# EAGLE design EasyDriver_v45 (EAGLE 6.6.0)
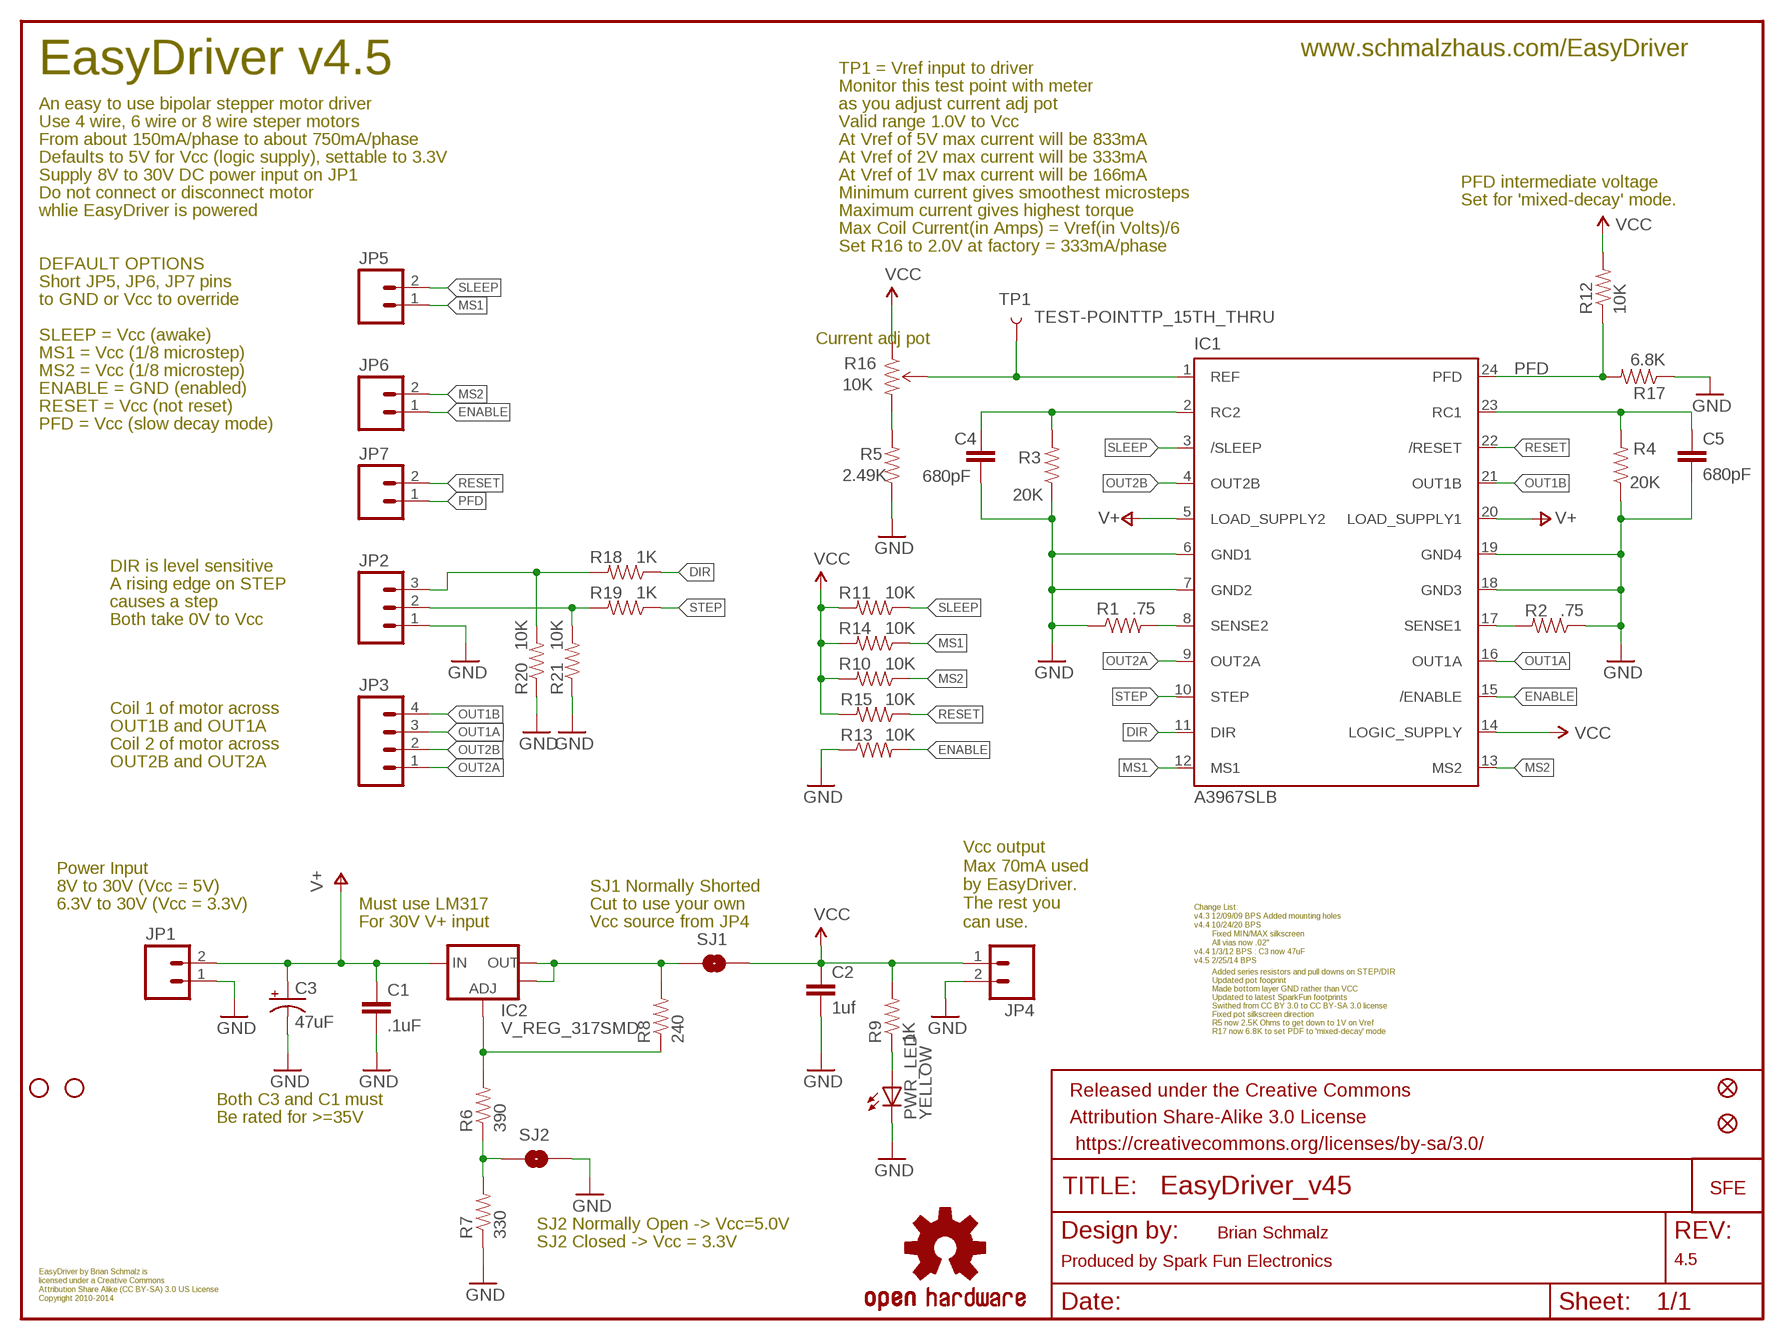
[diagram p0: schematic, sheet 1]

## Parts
C1  .1uF  CAP0603-CAP  [0603-CAP]
C2  1uf  CAP0603-CAP  [0603-CAP]
C3  47uF  CPOL-USD  [PANASONIC_D]
C4  680pF  CAP0603-CAP  [0603-CAP]
C5  680pF  CAP0603-CAP  [0603-CAP]
FID1  FIDUCIAL1X2  [FIDUCIAL-1X2]
FID2  FIDUCIAL1X2  [FIDUCIAL-1X2]
FRAME2  FRAME-LETTER  [CREATIVE_COMMONS]
IC1  A3967SLB  [SO24W]
IC2  V_REG_317SMD  [SOT223]
JP1  M021X02_NO_SILK  [1X02_NO_SILK]
JP2  M031X03_NO_SILK  [1X03_NO_SILK]
JP3  M041X04_NO_SILK  [1X04_NO_SILK]
JP4  M021X02_NO_SILK  [1X02_NO_SILK]
JP5  M021X02_NO_SILK  [1X02_NO_SILK]
JP6  M021X02_NO_SILK  [1X02_NO_SILK]
JP7  M021X02_NO_SILK  [1X02_NO_SILK]
JP8  STAND-OFF  [STAND-OFF]
JP9  STAND-OFF  [STAND-OFF]
LOGO1  OSHW-LOGOS  [OSHW-LOGO-S]
PWR_LED  YELLOW  LED-YELLOW0603  [LED-0603]
R1  .75  RESISTOR0805-RES  [0805]
R2  .75  RESISTOR0805-RES  [0805]
R3  20K  RESISTOR0603  [0603-RES]
R4  20K  RESISTOR0603  [0603-RES]
R5  2.49K  RESISTOR0603  [0603-RES]
R6  390  RESISTOR0603  [0603-RES]
R7  330  RESISTOR0603  [0603-RES]
R8  240  RESISTOR0603  [0603-RES]
R9  1K  RESISTOR0603  [0603-RES]
R10  10K  RESISTOR0603  [0603-RES]
R11  10K  RESISTOR0603  [0603-RES]
R12  10K  RESISTOR0603  [0603-RES]
R13  10K  RESISTOR0603  [0603-RES]
R14  10K  RESISTOR0603  [0603-RES]
R15  10K  RESISTOR0603  [0603-RES]
R16  10K  TRIMPOT3MM-2  [TRIMPOT-3MM-2]
R17  6.8K  RESISTOR0603  [0603-RES]
R18  1K  RESISTOR0603  [0603-RES]
R19  1K  RESISTOR0603  [0603-RES]
R20  10K  RESISTOR0603  [0603-RES]
R21  10K  RESISTOR0603  [0603-RES]
SJ1  SOLDERJUMPERTRACE  [SJ_2S-TRACE]
SJ2  SOLDERJUMPERNO  [SJ_2S-NO]
TP1  TEST-POINTTP_15TH_THRU  [TP_15TH]
U$2  LOGO-SFENEW  [SFE-NEW-WEBLOGO]

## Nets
5V_ALT: IC2.2(OUT) IC2.4(OUT) R8.2 SJ1.1
DIR: IC1.11(DIR) R18.1
DIR_IN: JP2.3 R18.2 R20.2
ENABLE: IC1.15(/ENABLE) JP6.1 R13.2
GND: C1.2 C2.2 C3.- C4.2 C5.2 IC1.6(GND1) IC1.7(GND2) IC1.18(GND3) IC1.19(GND4) JP1.1 JP2.1 JP4.2 PWR_LED.C R1.1 R2.1 R3.1 R4.1 R5.1 R7.1 R13.1 R17.1 R20.1 R21.1 SJ2.2
MS1: IC1.12(MS1) JP5.1 R14.1
MS2: IC1.13(MS2) JP6.2 R10.1
N$1: IC1.8(SENSE2) R1.2
N$2: PWR_LED.A R9.1
N$3: IC1.17(SENSE1) R2.2
N$4: R6.1 R7.2 SJ2.1
N$5: C4.1 IC1.2(RC2) R3.2
N$6: IC2.1(ADJ) R6.2 R8.1
N$7: C5.1 IC1.23(RC1) R4.2
N$11: R5.2 R16.3(CW)
OUT1A: IC1.16(OUT1A) JP3.3
OUT1B: IC1.21(OUT1B) JP3.4
OUT2A: IC1.9(OUT2A) JP3.1
OUT2B: IC1.4(OUT2B) JP3.2
PFD: IC1.24(PFD) JP7.1 R12.1 R17.2
RESET: IC1.22(/RESET) JP7.2 R15.1
SLEEP: IC1.3(/SLEEP) JP5.2 R11.1
STEP: IC1.10(STEP) R19.1
STEP_IN: JP2.2 R19.2 R21.2
V+: C1.1 C3.+ IC1.5(LOAD_SUPPLY2) IC1.20(LOAD_SUPPLY1) IC2.3(IN) JP1.2
VCC: C2.1 IC1.14(LOGIC_SUPPLY) JP4.1 R9.2 R10.2 R11.2 R12.2 R14.2 R15.2 R16.1(CCW) SJ1.2
VREF: IC1.1(REF) R16.2(WIPER) TP1.P$1

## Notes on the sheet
- www.schmalzhaus.com/EasyDriver
- EasyDriver v4.5 | TP1 = Vref input to driver
- Monitor this test point with meter
- An easy to use bipolar stepper motor driver | as you adjust current adj pot
- Use 4 wire, 6 wire or 8 wire steper motors | Valid range 1.0V to Vcc
- From about 150mA/phase to about 750mA/phase | At Vref of 5V max current will be 833mA
- Defaults to 5V for Vcc (logic supply), settable to 3.3V | At Vref of 2V max current will be 333mA
- Supply 8V to 30V DC power input on JP1 | At Vref of 1V max current will be 166mA
- PFD intermediate voltage
- Do not connect or disconnect motor | Minimum current gives smoothest microsteps
- Set for 'mixed-decay' mode.
- whlie EasyDriver is powered | Maximum current gives highest torque
- Max Coil Current(in Amps) = Vref(in Volts)/6
- Set R16 to 2.0V at factory = 333mA/phase
- DEFAULT OPTIONS
- Short JP5, JP6, JP7 pins
- to GND or Vcc to override
- SLEEP = Vcc (awake) | Current adj pot
- MS1 = Vcc (1/8 microstep)
- MS2 = Vcc (1/8 microstep)
- ENABLE = GND (enabled)
- RESET = Vcc (not reset)
- PFD = Vcc (slow decay mode)
- DIR is level sensitive
- A rising edge on STEP
- causes a step
- Both take 0V to Vcc
- Coil 1 of motor across
- OUT1B and OUT1A
- Coil 2 of motor across
- OUT2B and OUT2A
- Power Input
- 8V to 30V (Vcc = 5V) | SJ1 Normally Shorted
- 6.3V to 30V (Vcc = 3.3V) | Must use LM317 | Cut to use your own | Change List:
- v4.3 12/09/09 BPS Added mounting holes
- For 30V V+ input | Vcc source from JP4
- Vcc output
  Max 70mA used 
  by EasyDriver.
  The rest you 
  can use.
- v4.4 10/24/20 BPS
- Fixed MIN/MAX silkscreen
- All vias now .02"
- v4.4 1/3/12 BPS : C3 now 47uF
- v4.5 2/25/14 BPS
- Added series resistors and pull downs on STEP/DIR
  Updated pot fooprint
  Made bottom layer GND rather than VCC
  Updated to latest SparkFun footprints
  Swithed from CC BY 3.0 to CC BY-SA 3.0 license
  Fixed pot silkscreen direction
  R5 now 2.5K Ohms to get down to 1V on Vref
  R17 now 6.8K to set PDF to 'mixed-decay' mode
- Both C3 and C1 must
- Be rated for >=35V
- SJ2 Normally Open -> Vcc=5.0V
- Brian Schmalz
- SJ2 Closed -> Vcc = 3.3V
- Produced by Spark Fun Electronics | 4.5
- EasyDriver by Brian Schmalz is
- licensed under a Creative Commons
- Attribution Share Alike (CC BY-SA) 3.0 US License
- Copyright 2010-2014

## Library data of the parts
C1 C2 C4 C5 = SparkFun-Capacitors:CAP: Capacitor
C3 = rcl:CPOL-US: POLARIZED CAPACITOR, American symbol
FID1 FID2 = SparkFun-Aesthetics:FIDUCIAL: Fiducial Alignment Points
FRAME2 = SparkFun-Retired:FRAME-LETTER: Schematic Frame
IC1 = Allegro:A3967SLB: ANALOG DEVICES
IC2 = SparkFun03_30_09:V_REG_317: Voltage Regulator Standard LM317 adjustable voltage regulator. AOI (Adjust Output Input). Google 'LM317 Calculator' for easy to use app to get the two resistor values needed. 240/720 for 5V output. 240/390 for 3.3V output. Spark Fun Electronics SKU : COM-00527
JP1 JP4-JP7 = SparkFun:M02: Header 2
JP2 = SparkFun:M03: Header 3 Standard 3-pin 0.1" header. Use with straight break away headers (SKU : PRT-00116), right angle break away headers (PRT-00553), swiss pins (PRT-00743), machine pins (PRT-00117), and female headers (PRT-00115). Molex polarized connector foot print use with SKU : PRT-08232 with associated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
JP3 = SparkFun:M04: Header 4 Standard 4-pin 0.1" header. Use with straight break away headers (SKU : PRT-00116), right angle break away headers (PRT-00553), swiss pins (PRT-00743), machine pins (PRT-00117), and female headers (PRT-00115). Molex polarized connector foot print use with SKU : PRT-08231 with associated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
JP8 JP9 = SparkFun-7-28-09:STAND-OFF: Stand Off
LOGO1 = SparkFun-Aesthetics:OSHW-LOGO: Open Source Hardware Logo This logo indicates the piece of hardware it is found on incorporates a OSHW license and/or adheres to the definition of open source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
PWR_LED = SparkFun-LED:LED-YELLOW: Yellow SMD LEDs; PROD_ID: DIO-09003
R1-R15 R17-R21 = SparkFun-Resistors:RESISTOR: Resistor
R16 = SparkFun-Electromechanical:TRIMPOT: Various small potentiometers for "set-and-forget" applications
SJ1 SJ2 = SparkFun03_30_09:SOLDERJUMPER: Solder Jumper
TP1 = SparkFun-Passives:TEST-POINT: Bare copper test points for troubleshooting or ICT
U$2 = SparkFun:LOGO-SFE: Spark Fun Electronics PCB Logo

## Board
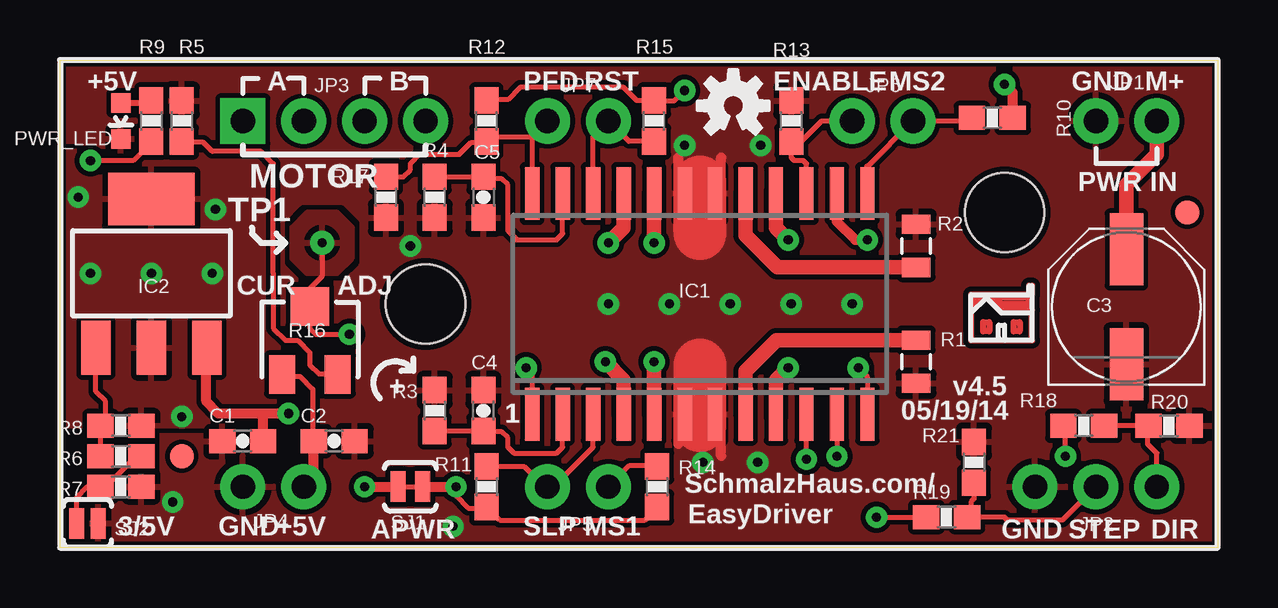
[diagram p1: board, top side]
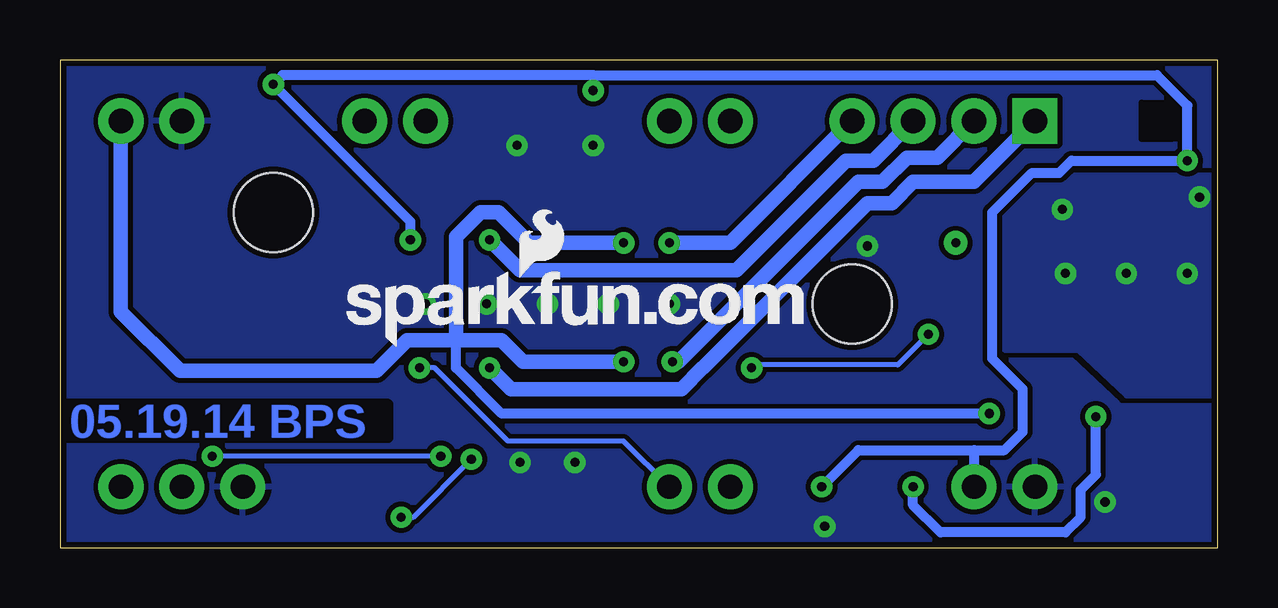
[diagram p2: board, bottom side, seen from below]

Size 48.26 x 20.32 mm. Coordinates in mm from the lower left corner, seen from the top.
Outline: 0,0 0,20.32 48.26,20.32 48.26,0 0,0
Copper layers (1*16): Top 0.035mm / dielectric 1.5mm / Bottom 0.035mm
Design rules "GoldPhoenix_8and8": minimum track width 7mil, minimum drill 15mil, track to track 8mil, track to pad 8mil, pad to pad 8mil, via to via 8mil, smd to smd 8mil, copper to edge 10mil, drill to drill 8mil, minimum pad ring 12mil, minimum via ring 10mil, stop-mask expansion 4mil, vias tented up to drill 25mil, thermal gap 10mil
bRestrict: area 1.9,17 to 3.2,18.5

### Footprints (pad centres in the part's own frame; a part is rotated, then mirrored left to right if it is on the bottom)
0603-CAP = smd 1.1 x 1: 1 -0.85,0; 2 0.85,0
PANASONIC_D = smd 3 x 1.4: + 2.4,0; - -2.4,0
FIDUCIAL-1X2 = smd 1 x 1: 1 0,0
SO24W = smd 0.6 x 2.2: 1 -6.985,-4.6; 2 -5.715,-4.6; 3 -4.445,-4.6; 4 -3.175,-4.6; 5 -1.905,-4.6; 6 -0.635,-4.6; 7 0.635,-4.6; 8 1.905,-4.6; 9 3.175,-4.6; 10 4.445,-4.6; 11 5.715,-4.6; 12 6.985,-4.6; 13 6.985,4.6; 14 5.715,4.6; 15 4.445,4.6; 16 3.175,4.6; 17 1.905,4.6; 18 0.635,4.6; 19 -0.635,4.6; 20 -1.905,4.6; 21 -3.175,4.6; 22 -4.445,4.6; 23 -5.715,4.6; 24 -6.985,4.6
SOT223 = smd 1.219 x 2.235: 1 -2.311,-3.099; 2 0,-3.099; 3 2.311,-3.099 | smd 3.6 x 2.2: 4 0,3.099
1X02_NO_SILK = drill 1.016 pad 1.88: 1 0,0; 2 2.54,0
1X03_NO_SILK = drill 1.016 pad 1.88: 1 0,0; 2 2.54,0; 3 5.08,0
1X04_NO_SILK = drill 1.016 pad 1.88 square: 1 0,0 | drill 1.016 pad 1.88: 2 2.54,0; 3 5.08,0; 4 7.62,0
STAND-OFF = hole 3.302: 0,0
LED-0603 = smd 0.8 x 0.8: A 0,-0.75; C 0,0.75
0805 = smd 0.8 x 1.2: 1 -0.9,0; 2 0.9,0
0603-RES = smd 1.1 x 1: 1 -0.85,0; 2 0.85,0
TRIMPOT-3MM-2 = smd 1.092 x 1.6: 1 -1.155,-1.421; 3 1.155,-1.421 | smd 1.6 x 1.6: 2 0,1.421
SJ_2S-TRACE = smd 0.635 x 1.27: 1 -0.508,0; 2 0.508,0
SJ_2S-NO = smd 0.635 x 1.27: 1 -0.45,0; 2 0.45,0
TP_15TH = drill 0.381 pad 0.61: P$1 0,0

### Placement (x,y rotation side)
C1  7.62,4.45 180 top
C2  11.43,4.45 0 top
C3  44.45,10.03 90 top
C4  17.65,5.71 90 top
C5  17.65,14.61 270 top
FID1  46.99,13.97 0 top
FID2  5.08,3.81 0 top
FRAME2  not placed on the board
IC1  26.67,10.16 0 top
IC2  3.81,11.43 0 top
JP1  43.18,17.78 0 top
JP2  40.64,2.54 0 top
JP3  7.62,17.78 0 top
JP4  10.16,2.54 180 top
JP5  22.86,2.54 180 top
JP6  33.02,17.78 0 top
JP7  20.32,17.78 0 top
JP8  39.37,13.97 0 top
JP9  15.24,10.16 0 top
LOGO1  28.07,18.41 0 top
PWR_LED  2.54,17.78 180 top
R1  35.69,7.75 90 top
R2  35.69,12.57 270 top
R3  15.62,5.71 270 top
R4  15.62,14.61 90 top
R5  5.08,17.78 270 top
R6  2.54,3.81 180 top
R7  2.54,2.54 180 top
R8  2.54,5.08 0 top
R9  3.81,17.78 270 top
R10  38.86,17.91 0 top
R11  17.78,2.54 270 top
R12  17.78,17.78 90 top
R13  30.48,17.78 270 top
R14  24.89,2.54 270 top
R15  24.77,17.78 90 top
R16  10.41,8.64 0 top
R17  13.59,14.61 90 top
R18  42.67,5.08 0 top
R19  36.96,1.27 0 top
R20  46.23,5.08 180 top
R21  38.1,3.56 270 top
SJ1  14.61,2.54 0 top
SJ2  1.14,1.02 0 top
TP1  10.92,12.7 0 top
U$1  [SCHMALZHAUS_SMALL]  39.24,8.64 0 top
U$2  36.32,8.38 0 bottom

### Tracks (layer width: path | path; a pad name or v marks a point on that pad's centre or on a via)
5V_ALT  (via drill 0.38)
  Top 0.254: R8.2 3.81,5.08
  Top 0.406: v12.7,2.54 SJ1.1
  Bottom 0.406: v5.08,5.46 5.08,3.05 5.71,2.41 5.71,1.27 6.35,0.64 11.56,0.64 12.7,1.78 v12.7,2.54
  other vias: 1.27,11.43 3.81,11.43 6.35,11.43 6.48,14.1 0.76,14.61
  pour Top (rank 2): 0,5.08 0,16.51 10.16,16.51 10.16,5.08
  pour Bottom (rank 2): 0,15.49 7.49,15.49 8.89,13.97 8.89,8.26 5.84,8.26 3.81,6.35 0,6.35
DIR  (via drill 0.38)
  Top 0.203: IC1.11 v32.38,3.81 | v41.91,3.81 41.91,4.99 R18.1
  Bottom 0.203: v32.38,3.81 v41.91,3.81
DIR_IN
  Top 0.203: JP2.3 45.72,3.94 45.34,4.32 45.34,5.04 R20.2 R18.2
ENABLE
  Top 0.203: IC1.15 31.11,16 30.99,16.13 30.61,16.13 30.48,16.26 R13.2 30.9,16.93 31.75,17.78 JP6.1
GND  (via drill 0.38)
  Top 0.203: 25.78,6.99 26.29,6.99 26.67,7.37
  Top 0.406: 27.56,3.81 27.56,7.24 | 27.56,13.21 27.56,16.26 | 25.78,13.21 25.78,16.26 | 25.78,4.32 25.78,6.99
  Top 2.184: 26.67,13.08 26.67,15.24 | 26.67,5.08 26.67,7.37 26.67,7.62
  other vias: 25.4,10.16 27.94,10.16 22.86,10.16 30.48,10.16 33.02,10.16 4.7,1.91 14.61,12.57 16.38,0.89 26.8,3.56 29.08,3.56 26.04,16.76 29.21,16.76
  pour Top (rank 3): 0,0 0,5.08 0,20.32 48.26,20.32 48.26,0
  pour Bottom (rank 3): 15.24,17.78 17.65,15.24 17.78,15.37 17.65,15.37
  pour Bottom (rank 4): 0,0 0,20.32 48.26,20.32 48.26,0
MS1  (via drill 0.38)
  Top 0.203: IC1.12 33.66,7.11 v33.27,7.49 | 23.51,3.19 JP5.1 23.75,3.43 24.85,3.43 R14.1
  Bottom 0.203: v33.27,7.49 32.64,7.49 29.59,4.45 24.77,4.45 JP5.1
MS2
  Top 0.203: 33.66,15.88 JP6.2 37.88,17.78 R10.1
  Top 0.254: IC1.13 33.66,15.88
N$1
  Top 0.406: 35.31,8.64 35.69,8.64 R1.2
  Top 0.61: IC1.8 28.57,7.34 29.87,8.64 35.31,8.64
N$2
  Top 0.254: PWR_LED.A 3.81,18.53 R9.1
N$3
  Top 0.406: 35.31,11.68 35.69,11.68 R2.2
  Top 0.61: IC1.17 28.57,13.02 29.91,11.68 35.31,11.68
N$4
  Top 0.203: SJ2.1 0.69,2.09 1.14,2.54 R7.2 1.91,2.54 2.92,3.56 3.14,3.56 R6.1
N$5
  Top 0.203: R3.2 C4.1 17.69,4.83 18.41,4.83 18.67,4.57 18.67,4.19 18.92,3.94 20.7,3.94 20.95,4.19 IC1.2
N$6
  Top 0.203: R6.2 R8.1 | 1.91,5.08 1.91,6.1 1.5,6.5 IC2.1
  Top 0.406: 1.27,8.1 1.5,8.1 IC2.1 | R8.1 1.91,5.08
N$7
  Top 0.203: IC1.23 20.95,13.08 20.7,12.83 19.05,12.83 18.67,13.21 18.67,15.11 18.41,15.37 17.74,15.37 C5.1 R4.2
N$11
  Top 0.203: R5.2 5.12,16.89 5.97,16.89 6.35,16.51 8.38,16.51 8.89,16 8.89,11.43 8.89,9.14 9.4,8.64 9.91,8.64 10.41,8.13 10.41,7.62 10.79,7.24 11.54,7.24 R16.3
OUT1A  (via drill 0.38)
  Top 0.406: IC1.16 29.94,14.76
  Top 0.61: 29.84,14.86 IC1.16 29.84,13.34 v30.35,12.83
  Bottom 0.61: v30.35,12.83 29.08,11.56 20.07,11.56 15.49,16.13 14.35,16.13 JP3.3
OUT1B  (via drill 0.38)
  Top 0.61: v22.86,12.7 23.5,13.34 IC1.21
  Bottom 0.61: v22.86,12.7 20.32,12.7 JP3.4
OUT2A  (via drill 0.38)
  Top 0.406: IC1.9 29.75,5.56
  Top 0.61: 29.84,5.46 IC1.9 29.84,6.99 v30.35,7.49
  Bottom 0.406: 21.46,7.49 21.47,7.49
  Bottom 0.61: 21.46,7.49 14.61,14.35 13.59,14.35 12.7,15.24 10.16,15.24 JP3.1 | v30.35,7.49 29.46,6.6 22.36,6.6 21.47,7.49
OUT2B  (via drill 0.38)
  Top 0.61: v22.73,7.75 23.5,6.99 IC1.4
  Bottom 0.61: JP3.2 11.68,16.26 12.95,16.26 13.97,15.24 14.99,15.24 22.48,7.75 v22.73,7.75
PFD
  Top 0.203: 19.68,17.14 IC1.24 | 17.8,17.13 19.67,17.13 JP7.1 | 17.8,17.13 17.8,16.95 R12.1 17.74,16.89 17.14,16.89 16.64,16.38 14.99,16.38 14.61,16 14.61,15.75 14.31,15.46 R17.2 | 17.8,17.13 17.78,17.13 17.77,17.14
  Top 0.254: IC1.24 19.68,14.73 | 19.67,17.13 19.68,17.14
RESET
  Top 0.203: IC1.22 22.23,17.14 JP7.2 23.71,16.93 R15.1
SLEEP
  Top 0.203: IC1.3 22.23,4.19 20.57,2.54 JP5.2 20.19,2.54 19.34,3.39 R11.1
  Top 0.305: IC1.3 22.23,5.59
STEP  (via drill 0.38)
  Top 0.203: v31.11,3.68 IC1.10 | v34.04,1.27 R19.1
  Bottom 0.203: v34.04,1.27 33.53,1.27 v31.11,3.68
STEP_IN
  Top 0.203: JP2.2 41.78,1.14 39.5,1.14 39.37,1.27 R19.2 37.97,1.44 37.97,1.91 38.1,2.03 R21.2
V+  (via drill 0.38)
  Top 0.203: 8.47,5.55 8.51,5.59
  Top 0.406: IC2.3 6.12,8.31 6.1,8.31 6.1,6.1 6.6,5.59 8.51,5.59 v9.53,5.59 | C1.1 8.47,5.55
  Top 0.61: v24.77,12.7 IC1.20 | v24.77,7.75 IC1.5 | C3.+ 44.45,15.11 45.72,16.38 JP1.2
  Bottom 0.406: 31.75,8.64 31.75,7.49 29.84,5.59 v9.53,5.59
  Bottom 0.61: v24.77,7.75 28.96,7.75 29.84,8.64 31.75,8.64 | 31.75,8.64 33.78,8.64 35.05,7.37 43.25,7.37 45.72,9.83 JP1.2 | v24.77,12.7 28.7,12.7 29.97,13.97 30.73,13.97 31.75,12.95 31.75,8.64
VCC  (via drill 0.38)
  Top 0.203: 24.93,1.69 24.38,1.14 18.33,1.14 R11.2 17.74,1.65 17.02,1.65 16.51,2.16 v16.51,2.54 | R9.2 3.81,16.89 3.05,16.13 v1.27,16.13 | C2.1 10.54,4.48 10.54,6.6 10.03,7.11 9.36,7.11 R16.1 | v26.04,19.05 25.61,18.63 R15.2 24.04,18.63 23.5,19.18 19.18,19.18 18.67,18.67 17.82,18.67 R12.2
  Top 0.254: 24.93,1.69 R14.2
  Top 0.406: IC1.14 32.38,13.59 33.15,12.83 v33.66,12.83 | SJ1.2 v16.51,2.54 | C2.1 10.58,2.96 JP4.1 | R10.2 39.71,18.96 v39.37,19.3
  Bottom 0.203: v33.66,12.83 33.66,12.95 | JP4.1 | v26.04,19.05 26.04,19.68
  Bottom 0.406: 33.66,12.95 33.66,13.59 v39.37,19.3 38.99,19.68 38.35,19.68 26.04,19.68 2.54,19.68 1.27,18.41 v1.27,16.13 6.1,16.13 6.6,15.62 7.75,15.62 9.4,13.97 9.4,7.87 8.13,6.6 8.13,4.83 8.89,4.06 10.16,4.06 | v16.51,2.54 14.99,4.06 10.16,4.06 | 10.16,4.06 JP4.1
VREF  (via drill 0.38)
  Top 0.203: IC1.1 19.68,7.24 v19.43,7.49 | v12.06,8.89 10.67,8.89 10.41,9.14 R16.2 10.41,10.79 10.92,11.3 TP1.P$1
  Bottom 0.203: 19.3,7.62 13.34,7.62 v12.06,8.89
  Bottom 0.254: 19.3,7.62 v19.43,7.49
  pour Top: 11.56,13.97 10.29,13.97 9.65,13.34 9.65,12.06 10.29,11.43 11.56,11.43 12.19,12.06 12.19,13.34

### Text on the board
Bottom: 05.19.14 BPS
tPlace: +5V | A | B | PFD | RST | ENABLE | MS2 | GND | M+ | MOTOR | PWR IN | TP1 | CUR | ADJ | + | v4.5 | 1 | 05/19/14 | SchmalzHaus.com/ | 3/5V | GND | +5V | SLP | MS1 | EasyDriver | APWR | GND | STEP | DIR
tDocu: Brian Schmalz | Produced by SparkFun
